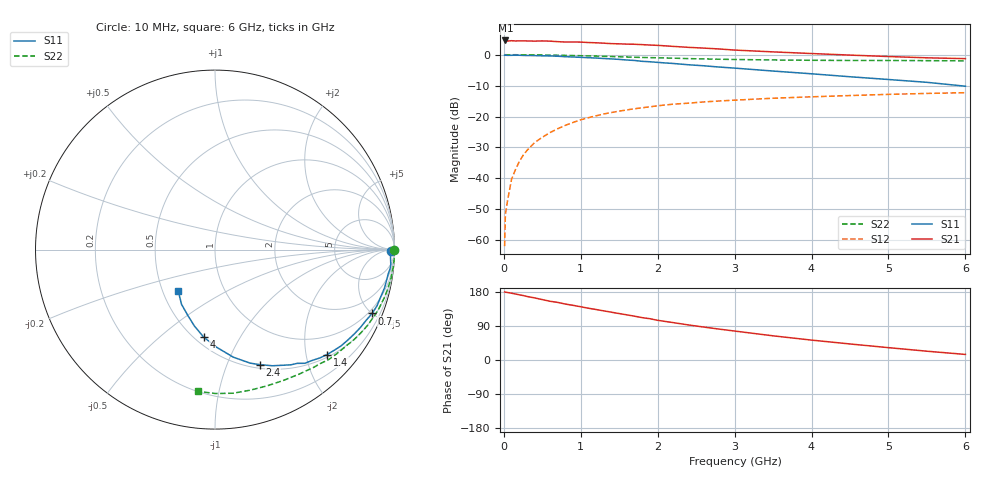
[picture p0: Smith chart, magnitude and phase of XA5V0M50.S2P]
! SIEMENS Discrete & RF Semiconductors
! BFY180
! Si NPN RF Bipolar Junction Transistor in MICRO-X
! VCE = 5 V  IC = 0.5 mA
! Common Emitter S-Parameters:  May  1997
# GHz  S  MA  R  50
!  f  S11  S21  S12  S22
! GHz  MAG  ANG  MAG  ANG  MAG  ANG  MAG  ANG
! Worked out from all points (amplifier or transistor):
!   36 points, 10 MHz to 6 GHz, reference 50 ohm
!   highest |S21| = 4.6 dB at 20 MHz (marker M1)
!   |S21| within 3 dB of that: start of sweep to 2.938 GHz
!   unconditionally stable (mu >= 1): 5.865 GHz to end of sweep
!   at 250 MHz: K = 0.06, MSG = 18.5 dB, |S12| = -32.6 dB
!   at 1.4 GHz: K = 0.38, MSG = 11.1 dB, |S12| = -18.7 dB
!   at 6 GHz: K = 1.00, MAG = 5.1 dB, |S12| = -12.3 dB
!   S11 on the Smith chart (normalised r, x): 10 MHz: open; 700 MHz: 0.75, -5.01; 1.4 GHz: 0.56, -2.42; 2.4 GHz: 0.54, -1.32; 4 GHz: 0.55, -0.71; 6 GHz: 0.60, -0.31
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0.01  0.9824 -0.4  1.688 179.6  0.0008 90.5  0.9995 -0.1
0.02  0.9823 -0.7  1.701 179.0  0.0026 90.0  0.9995 -0.5
0.05  0.9777 -1.5  1.666 178.1  0.0045 83.0  0.9986 -1.1
0.1  0.9795 -3.0  1.686 176.2  0.0096 89.1  0.9988 -2.3
0.2  0.9811 -6.3  1.676 172.0  0.0186 85.2  0.9975 -4.5
0.3  0.9719 -9.6  1.671 167.7  0.0282 82.5  0.9952 -6.7
0.4  0.9685 -12.7  1.66 163.9  0.0379 80.2  0.994 -8.9
0.6  0.9552 -19.2  1.658 155.0  0.055 75.0  0.9857 -13.4
0.7  0.945 -22.1  1.626 152.0  0.0635 72.4  0.9813 -15.6
0.9  0.9187 -28.3  1.609 144.2  0.0802 67.5  0.9703 -19.9
1.1  0.8951 -34.3  1.574 136.6  0.0958 62.9  0.9562 -24.0
1.4  0.8554 -43.1  1.511 126.1  0.1161 56.2  0.9343 -30.1
1.8  0.7815 -54.2  1.456 111.7  0.1388 48.8  0.9033 -37.3
2  0.7512 -59.0  1.417 104.7  0.1493 45.1  0.8921 -40.7
2.2  0.7219 -63.7  1.364 98.7  0.1584 41.5  0.8806 -44.2
2.4  0.6878 -68.7  1.316 92.5  0.1646 38.5  0.8643 -47.3
2.8  0.6317 -76.7  1.239 81.5  0.1786 33.1  0.8449 -53.1
3.5  0.5443 -89.0  1.111 63.8  0.1977 24.8  0.8224 -62.5
4  0.4915 -97.4  1.045 52.5  0.2085 19.5  0.8125 -69.2
4.5  0.4402 -105.2  0.986 42.3  0.2185 14.8  0.8073 -75.9
5.5  0.3576 -121.4  0.891 23.2  0.2365 5.6  0.8019 -89.8
6  0.3095 -131.3  0.864 14.7  0.2431 0.9  0.7955 -96.7
